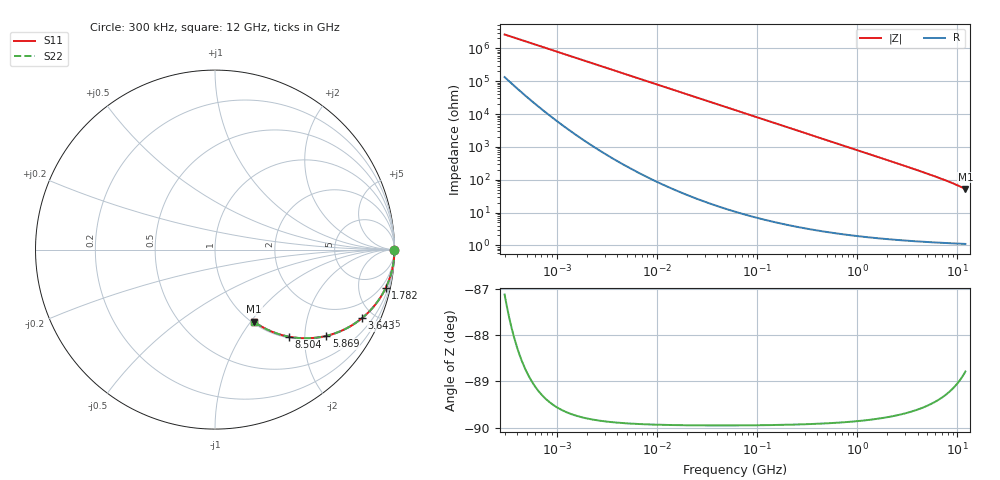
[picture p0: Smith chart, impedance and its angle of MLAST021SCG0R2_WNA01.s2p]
! MLAST021SCG0R2_WNA01  S-PARAMETER MODEL  ( General Type )
! Model Generated by TAIYO YUDEN Corporation (http://www.ty-top.com)
! Version 1.0
! TAIYO YUDEN Control No. 220901
! Copyright(c) 2022 TAIYO YUDEN CO.,LTD. All Rights Reserved.
! Product Description (link to TY-COMPAS)
! https://ds.yuden.co.jp/TYCOMPAS/or/detail?pn=MLAST021SCG0R2BWNA01&u=M
! Products Name : Multilayer Ceramic Capacitors
! Characteristics :
!  Capacitance : 0.2 pF , Rated Voltage : 25V , TCC : CG / C0G
!  Case Size : 0.25 x 0.125 / 0.0098 x 0.0049 [mm/inch] , Thickness : 0.125 / 0.0049 [mm/inch]
!  (Conditions: Temperature = 25 degC , DC Bias Current/Voltage = 0A / 0V)
! External Node Assignments :
!  1  o---| |---o  2
! GND o---------o GND
! Frequency Range : 0.3MHz  -  12000MHz  [ 401 STEP ]
# MHz S RI R 50
! Freq[MHz].  S11 Real  S11 Imag  S21 Real  S21 Imag  S12 Real  S12 Imag  S22 Real  S22 Imag
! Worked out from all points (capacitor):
!   401 points, 300 kHz to 12 GHz, reference 50 ohm
!   read as one part in series: C = 201 fF near 316.3 kHz
!   lowest |Z| = 52 ohm at 12 GHz (marker M1)
!   S11 on the Smith chart (normalised r, x): 300 kHz: open; 1.782 GHz: 1.03, -8.85; 3.643 GHz: 1.03, -4.26; 5.869 GHz: 1.02, -2.56; 8.504 GHz: 1.02, -1.66; 12 GHz: 1.02, -1.04
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0.3  1 -3.78e-05  1.91e-06 3.78e-05  1.91e-06 3.78e-05  1 -3.78e-05
0.778586  1 -9.82e-05  1.06e-06 9.82e-05  1.06e-06 9.82e-05  1 -9.82e-05
0.842989  1 -0.000106  1.04e-06 0.000106  1.04e-06 0.000106  1 -0.000106
1.769972  1 -0.000224  9.21e-07 0.000224  9.21e-07 0.000224  1 -0.000224
10.44266  1 -0.00132  3.13e-06 0.00132  3.13e-06 0.00132  1 -0.00132
60  0.9999 -0.00758  6.35e-05 0.00758  6.35e-05 0.00758  0.9999 -0.00758
164.1901  0.9995 -0.0207  0.00045 0.0207  0.00045 0.0207  0.9995 -0.0207
353.9943  0.9979 -0.0446  0.00206 0.0446  0.00206 0.0446  0.9979 -0.0446
570.2811  0.9947 -0.0717  0.00529 0.0717  0.00529 0.0717  0.9947 -0.0717
871.3074  0.9878 -0.1088  0.0122 0.1088  0.0122 0.1088  0.9878 -0.1088
1262.535  0.9747 -0.1557  0.0253 0.1557  0.0253 0.1557  0.9747 -0.1557
1781.601  0.9507 -0.2147  0.0493 0.2147  0.0493 0.2147  0.9507 -0.2147
2088.533  0.9333 -0.2475  0.0667 0.2475  0.0667 0.2475  0.9333 -0.2475
2795.104  0.8857 -0.3157  0.1143 0.3157  0.1143 0.3157  0.8857 -0.3157
3642.919  0.818 -0.3827  0.182 0.3827  0.182 0.3827  0.818 -0.3827
4623.766  0.7318 -0.4392  0.2682 0.4392  0.2682 0.4392  0.7318 -0.4392
5868.704  0.6202 -0.4806  0.3798 0.4806  0.3798 0.4806  0.6202 -0.4806
7064.448  0.5188 -0.4939  0.4812 0.4939  0.4812 0.4939  0.5188 -0.4939
8503.825  0.4104 -0.485  0.5896 0.485  0.5896 0.485  0.4104 -0.485
9708.23  0.3331 -0.4633  0.6669 0.4633  0.6669 0.4633  0.3331 -0.4633
11083.22  0.2593 -0.4288  0.7407 0.4288  0.7407 0.4288  0.2593 -0.4288
12000  0.2179 -0.4024  0.7821 0.4024  0.7821 0.4024  0.2179 -0.4024
